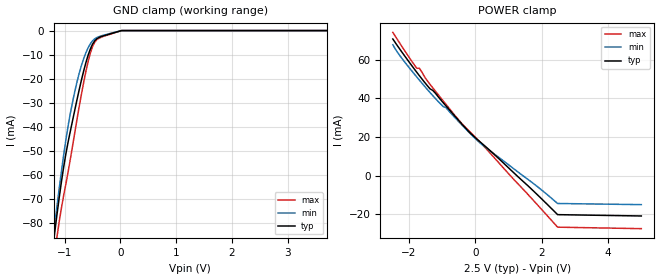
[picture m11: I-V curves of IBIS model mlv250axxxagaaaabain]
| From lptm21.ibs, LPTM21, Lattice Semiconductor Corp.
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|   Model mlv250axxxagaaaabain
[Model]   mlv250axxxagaaaabain
Model_type   Input
Polarity   Non-Inverting
Enable   Active-Low
Vinl =   1.1500V
Vinh =   1.3500V
C_comp   4.2000pF   3.8000pF   7.5000pF
[Temperature Range]   25.0000   0.1050k   -40.0000
[Voltage Range]   2.5000V   2.3800V   2.6300V
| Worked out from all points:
|   GND clamp passes 1 mA (typ) near -0.13 V on its own axis
[GND_clamp]
|Voltage   I(typ)   I(min)   I(max)
-2.5V     -559mA     -539.3mA   -577.6mA
-1.22V    -91.87mA   -88.8mA    -100.4mA
-1.18V    -84.23mA   -80.98mA   -92.97mA
-1.14V    -76.86mA   -73.36mA   -86.09mA
-1.02V    -57.03mA   -52.06mA   -68.84mA
-940mV    -46.52mA   -39.84mA   -58.98mA
-780mV    -28.85mA   -21.43mA   -37.05mA
-580mV    -10.26mA   -7.144mA   -12.89mA
-500mV    -5.622mA   -4.259mA   -6.605mA
-420mV    -3.366mA   -2.868mA   -3.715mA
20mV      0A         0A         0A
5V        0A         0A         0A
[POWER_clamp]
|Voltage   I(typ)   I(min)   I(max)
-2.48V    70.8mA     67.79mA    74.22mA
-2.24V    64.81mA    61.5mA     67.79mA
-1.76V    53.56mA    51.12mA    55.62mA
-1.68V    51.75mA    49.46mA    55.62mA
-1.36V    44.95mA    43.02mA    47.29mA
-1.2V     42.73mA    39.97mA    43.79mA
-960mV    37.69mA    35.72mA    38.61mA
-880mV    36.09mA    35.18mA    36.9mA
-480mV    28.21mA    27.66mA    28.47mA
0V        19.67mA    19.21mA    19.91mA
2.48V     -20.27mA   -14.48mA   -26.76mA
5V        -20.96mA   -15.08mA   -27.53mA
